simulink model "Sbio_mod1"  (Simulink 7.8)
settings: Solver=ode23t  StartTime=0.0  StopTime=0.5  MinStep=2.9e-4  RelTol=1e-2
PostLoadFcn:
  | openscopes;
undefined symbols (not defined in the file or in its folder): boitier, kg, m, N, porte, poussoir, rad, RootGround, RootPart, s, sigbuilder_block, STL
libraries: mblibv1 x22, fl_lib x16, elec_lib x9, nesl_utility x7

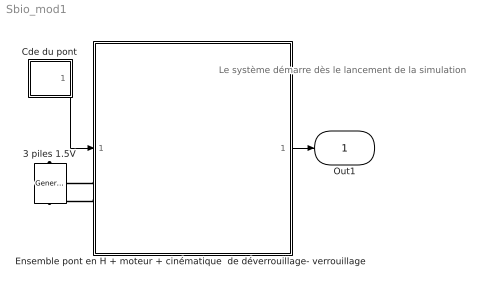
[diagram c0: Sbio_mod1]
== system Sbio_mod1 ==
  note: Le système démarre dès le lancement de la simulation
  3 piles 1.5V : elec_lib/Sources/Generic Battery  Vnom=4.5 V  R1=0.6 Ohm  prm_AH=1  AH=50 hr*A  AH0=50 hr*A  V1=11.5 V  AH1=25 hr*A  prm_R2=1  R2=2e+3 Ohm  LocalVarLogging=[]
  Cde du pont : Subsystem
  Ensemble pont en H + moteur + cinématique  de déverrouillage- verrouillage : Subsystem
  Out1 : Outport
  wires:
  Ensemble pont en H + moteur + cinématique  de déverrouillage- verrouillage/1(Sortie) -> Out1/1
  Cde du pont/1(Out1) -> Ensemble pont en H + moteur + cinématique  de déverrouillage- verrouillage/1(Cdes)
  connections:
  3 piles 1.5V/LConn1 -- Ensemble pont en H + moteur + cinématique  de déverrouillage- verrouillage/LConn1
  3 piles 1.5V/RConn1 -- Ensemble pont en H + moteur + cinématique  de déverrouillage- verrouillage/LConn2

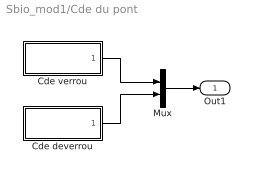
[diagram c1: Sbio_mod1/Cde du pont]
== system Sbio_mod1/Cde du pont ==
  Cde deverrou : Subsystem  Tag=STV Subsys  LoadFcn=sigbuilder_block('load');  StartFcn=sigbuilder_block('start');  StopFcn=sigbuilder_block('stop');  ClipboardFcn=sigbuilder_block('clipboard');
  Cde verrou : Subsystem  Tag=STV Subsys  LoadFcn=sigbuilder_block('load');  StartFcn=sigbuilder_block('start');  StopFcn=sigbuilder_block('stop');  ClipboardFcn=sigbuilder_block('clipboard');
  Mux : Mux  Inputs=2
  Out1 : Outport
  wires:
  Mux/1 -> Out1/1
  Cde verrou/1(Signal 1) -> Mux/1
  Cde deverrou/1(Signal 1) -> Mux/2

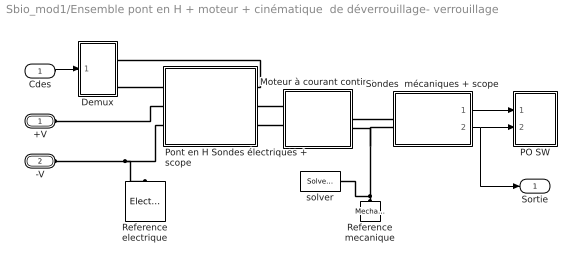
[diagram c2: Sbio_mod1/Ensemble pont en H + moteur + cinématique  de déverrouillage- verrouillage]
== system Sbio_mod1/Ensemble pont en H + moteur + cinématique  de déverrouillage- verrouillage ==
  Cdes : Inport
  Demux : Subsystem
  Moteur à courant continu : Subsystem
  PO SW : Subsystem
  Pont en H Sondes électriques + scope : Subsystem
  Reference electrique : fl_lib/Electrical/Electrical Elements/Electrical Reference  i_Log=off  LocalVarNames=|i  LocalVarDescs=|i  LocalVarLogging=0
  Reference mecanique : fl_lib/Mechanical/Rotational Elements/Mechanical Rotational Reference  t_Log=off  LocalVarNames=|t  LocalVarDescs=|t  LocalVarLogging=0
  Sondes  mécaniques + scope : Subsystem
  solver : nesl_utility/Solver Configuration  PhysicalDomain=network_engine_domain  LeftPortType=input  RightPortType=generic  SubClassName=solver  DoDC=off  ResidualTolerance=1e-9  UseLocalSolver=on  LocalSolverChoice=NE_BACKWARD_EULER_ADVANCER  LocalSolverSampleTime=3e-4  DoFixedCost=on  MaxNonlinIter=5  MaxModeIter=2  LinearAlgebra=Sparse  Accelerate=off  Profile=off  UseLocalSampling=off  DelaysMemoryBudget=1024
  +V : PMIOPort  Port=1  Side=Left
  -V : PMIOPort  Port=2  Side=Left
  Sortie : Outport
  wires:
  Sondes  mécaniques + scope/2(Out2) -> Sortie/1, PO SW/2(In2)
  Sondes  mécaniques + scope/1(Out1) -> PO SW/1(In1)
  Cdes/1 -> Demux/1(I1)
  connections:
  Pont en H Sondes électriques + scope/RConn2 -- +V/RConn1
  -V/RConn1 -- Reference electrique/LConn1 -- Pont en H Sondes électriques + scope/RConn3
  Reference mecanique/LConn1 -- Moteur à courant continu/RConn2 -- Sondes  mécaniques + scope/LConn2 -- solver/RConn1
  Moteur à courant continu/LConn1 -- Pont en H Sondes électriques + scope/LConn2
  Moteur à courant continu/LConn2 -- Pont en H Sondes électriques + scope/LConn3
  Moteur à courant continu/RConn1 -- Sondes  mécaniques + scope/LConn1
  Demux/RConn2 -- Pont en H Sondes électriques + scope/RConn1
  Demux/RConn1 -- Pont en H Sondes électriques + scope/LConn1

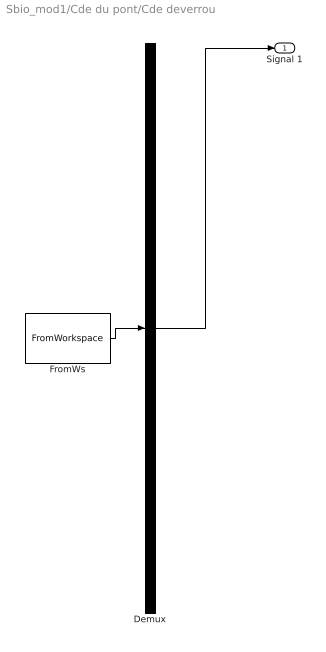
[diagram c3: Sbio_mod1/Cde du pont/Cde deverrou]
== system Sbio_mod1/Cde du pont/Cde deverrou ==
  Demux : Demux  Tag=STV Demux  Outputs=1
  FromWs : FromWorkspace  Tag=STV FromWs  VariableName=tuvar  SampleTime=0  SigBuilderData=DataTag0  VnvData=DataTag1
  Signal 1 : Outport  Tag=STV Outport
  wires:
  Demux/1 -> Signal 1/1
  FromWs/1 -> Demux/1

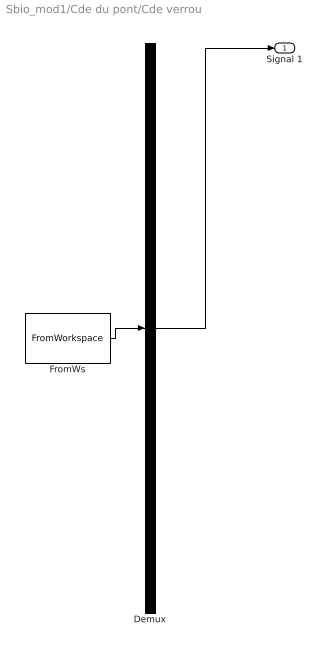
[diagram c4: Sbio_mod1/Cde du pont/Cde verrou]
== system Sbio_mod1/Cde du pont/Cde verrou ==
  Demux : Demux  Tag=STV Demux  Outputs=1
  FromWs : FromWorkspace  Tag=STV FromWs  VariableName=tuvar  SampleTime=0  SigBuilderData=DataTag2  VnvData=DataTag3
  Signal 1 : Outport  Tag=STV Outport
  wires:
  Demux/1 -> Signal 1/1
  FromWs/1 -> Demux/1

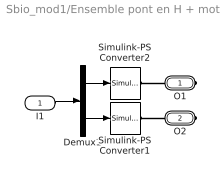
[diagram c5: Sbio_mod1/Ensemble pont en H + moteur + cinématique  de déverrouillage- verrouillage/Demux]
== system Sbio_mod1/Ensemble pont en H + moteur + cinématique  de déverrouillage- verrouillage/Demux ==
  I1 : Inport
  Demux1 : Demux  Outputs=2
  Simulink-PS Converter1 : nesl_utility/Simulink-PS Converter  PhysicalDomain=network_engine_domain  LeftPortType=input  RightPortType=output  SubClassName=ps_input  Unit=1  AffineConversion=off  InputFilterTimeConstant=.01  UdotUserProvided=0
  Simulink-PS Converter2 : nesl_utility/Simulink-PS Converter  PhysicalDomain=network_engine_domain  LeftPortType=input  RightPortType=output  SubClassName=ps_input  Unit=1  AffineConversion=off  InputFilterTimeConstant=.01  UdotUserProvided=0
  O1 : PMIOPort  Port=1  Side=Right
  O2 : PMIOPort  Port=2  Side=Right
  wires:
  Demux1/1 -> Simulink-PS Converter2/1
  Demux1/2 -> Simulink-PS Converter1/1
  I1/1 -> Demux1/1
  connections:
  O1/RConn1 -- Simulink-PS Converter2/RConn1
  O2/RConn1 -- Simulink-PS Converter1/RConn1

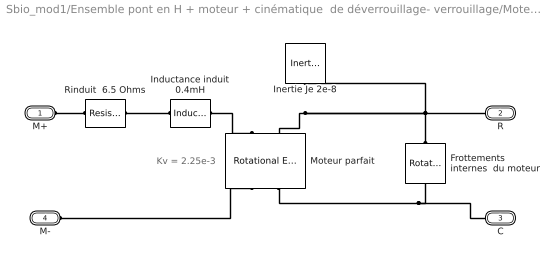
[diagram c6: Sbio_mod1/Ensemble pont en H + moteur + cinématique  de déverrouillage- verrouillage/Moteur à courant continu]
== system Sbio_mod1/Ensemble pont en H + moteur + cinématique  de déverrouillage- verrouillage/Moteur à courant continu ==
  note: Kv = 2.25e-3
  Frottements internes  du moteur : fl_lib/Mechanical/Rotational Elements/Rotational Friction  brkwy_trq=4e-5 N*m  Col_trq=4e-5 N*m  visc_coef=6e-8 N*m/(rad/s)  trans_coef=10 s/rad  vel_thr=1 rad/s  t_Log=off  w_Log=off  LocalVarNames=|t|w  LocalVarDescs=|t|w  LocalVarLogging=[0 0]
  Inductance induit 0.4mH : fl_lib/Electrical/Electrical Elements/Inductor  l=0.4 mH  i0=0 A  r=0 Ohm  g=1e-09 1/Ohm  i_Log=off  v_Log=off  i_L_Log=off  LocalVarNames=|current|voltage|power  LocalVarDescs=|Inductor current (A) |Voltage across inductor (V)|Power (W)  LocalVarLogging=[0 0 0]
  Inertie Je 2e-8 : fl_lib/Mechanical/Rotational Elements/Inertia  inertia=2e-8 kg*m^2  initial_velocity=0 rad/s  t_Log=off  LocalVarNames=|torque|velocity  LocalVarDescs=|Inertia torque (N*m)|Inertia absolute velocity (rad/s)  LocalVarLogging=[0 0]
  Moteur parfait : fl_lib/Electrical/Electrical Elements/Rotational Electromechanical Converter  K=2.25e-3 V/(rad/s)  i_Log=off  v_Log=off  t_Log=off  w_Log=off  LocalVarNames=|current|voltage|power|torque|speed  LocalVarDescs=|Current (A)|Voltage (V)|Power (W)|Torque (Nm)|Angular speed (rad/s)  LocalVarLogging=[0 0 0 0 0]
  Rinduit  6.5 Ohms : fl_lib/Electrical/Electrical Elements/Resistor  Tag=Factory Generic  R=6.5 Ohm  i_Log=off  v_Log=off  LocalVarNames=|current|voltage|power  LocalVarDescs=|Resistor current (A)|Voltage across resistor (V)|Power (W)  LocalVarLogging=[0 0 0]
  M+ : PMIOPort  Port=1  Side=Left
  R : PMIOPort  Port=2  Side=Right
  C : PMIOPort  Port=3  Side=Right
  M- : PMIOPort  Port=4  Side=Left
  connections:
  Moteur parfait/LConn1 -- Inductance induit 0.4mH/RConn1
  M-/RConn1 -- Moteur parfait/RConn1
  M+/RConn1 -- Rinduit  6.5 Ohms/LConn1
  Rinduit  6.5 Ohms/RConn1 -- Inductance induit 0.4mH/LConn1
  Moteur parfait/LConn2 -- Inertie Je 2e-8/LConn1 -- Frottements internes  du moteur/LConn1 -- R/RConn1
  Moteur parfait/RConn2 -- C/RConn1 -- Frottements internes  du moteur/RConn1

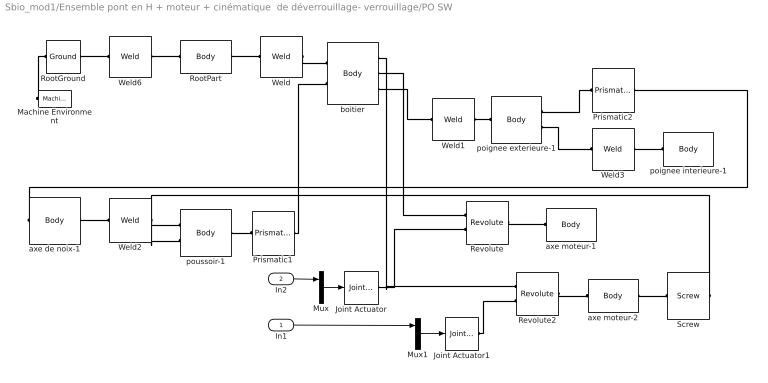
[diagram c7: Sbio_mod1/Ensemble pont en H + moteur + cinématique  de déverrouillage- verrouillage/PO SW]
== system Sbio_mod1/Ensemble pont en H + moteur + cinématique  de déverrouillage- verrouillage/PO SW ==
  In1 : Inport
  In2 : Inport  Port=2
  Joint Actuator : mblibv1/Sensors &  Actuators/Joint Actuator  UpdateFromCAD=off  PhysicalDomain=Mechanical  PortType=blob  ActuationStyle=Motion  AngleUnits=rev  ArcVelocityUnits=rad/s  ArcAccelerationUnits=rad/s^2  CoordPositionUnits=m  VelocityUnits=m/s  AccelerationUnits=m/s^2  ForceUnits=N  TorqueUnits=N*m  ActiveIO=on  Width=3  DialogClass=MechanicalActuatorBlock  Primitive=R1  ReferenceFrame=Absolute (World)
  Joint Actuator1 : mblibv1/Sensors &  Actuators/Joint Actuator  UpdateFromCAD=off  PhysicalDomain=Mechanical  PortType=blob  ActuationStyle=Motion  AngleUnits=rad  ArcVelocityUnits=rad/s  ArcAccelerationUnits=rad/s^2  CoordPositionUnits=m  VelocityUnits=m/s  AccelerationUnits=m/s^2  ForceUnits=N  TorqueUnits=N*m  ActiveIO=on  Width=3  DialogClass=MechanicalActuatorBlock  Primitive=R1  ReferenceFrame=Absolute (World)
  Machine Environment : mblibv1/Bodies/Machine Environment  PortType=env  PhysicalDomain=Mechanical  DialogTemplateClass=MECH.MachineEnvironment  SyncWhenCopied=off  Gravity=[0 -9.81 0]  GravityUnits=m/s^2  GravityAsSignal=off  Dimensionality=Auto-detect  AnalysisType=Forward dynamics  LinearAssemblyTolerance=1e1  LinearAssemblyToleranceUnits=m  AngularAssemblyTolerance=1e1  AngularAssemblyToleranceUnits=rad  ConstraintSolverType=Stabilizing  ConstraintRelTolerance=1e-4  ConstraintAbsTolerance=1e-4  UseRobustSingularityHandling=off  RedundancyAnalysisToleranceType=Specify tolerance  RedundancyAnalysisTolerance=1e-1  StatePerturbationType=Fixed  PerturbationSize=3e-4  VisualizeMachine=on  BodyVisualizationType=Use model default body geometries  BodyColorSelMode=Use model default  DefaultBodyColor=[1 0 0]
  Mux : Mux  Inputs=3
  Mux1 : Mux  Inputs=3
  Prismatic1 : mblibv1/Joints/Prismatic  LConnTagsString=__newl0  RConnTagsString=__newr0  UpdateFromCAD=off  NumSAPorts=0  CutJoint=off  MarkAsCut=off  Primitives=prismatic  PrimitiveProps=P1$World$[0 1 0]$prismatic  DialogClass=JointBlock  P1Axis=[0 1 0]
  Prismatic2 : mblibv1/Joints/Prismatic  LConnTagsString=__newl0  RConnTagsString=__newr0  UpdateFromCAD=off  NumSAPorts=0  CutJoint=off  MarkAsCut=off  Primitives=prismatic  PrimitiveProps=P1$World$[0 1 0]$prismatic  DialogClass=JointBlock  P1Axis=[0 1 0]
  Revolute : mblibv1/Joints/Revolute  LConnTagsString=__newl0|SA1  RConnTagsString=__newr0  UpdateFromCAD=on  PMImportedID=axe moteur-1:-:porte-1  NumSAPorts=1  CutJoint=off  MarkAsCut=off  Primitives=prismatic  PrimitiveProps=R1$World$[0,1,0]$revolute  DialogClass=JointBlock  R1Axis=[0,1,0]
  Revolute2 : mblibv1/Joints/Revolute  LConnTagsString=__newl0|SA1  RConnTagsString=__newr0  UpdateFromCAD=on  NumSAPorts=1  CutJoint=off  MarkAsCut=off  Primitives=prismatic  PrimitiveProps=R1$World$[0,1,0]$revolute  DialogClass=JointBlock  R1Axis=[0,1,0]
  RootGround : mblibv1/Bodies/Ground  UpdateFromCAD=on  PMImportedID=RootGround  LeftPortType=env  RightPortType=workingframe  PhysicalDomain=Mechanical  DialogClass=GroundBlock  CoordPosition=[-0.0761581,-0.00065379,-0.00321688]  CoordPositionUnits=m  StateVectorMgrId=0  MachineId=[1 0]  ShowEnvPort=on
  RootPart : mblibv1/Bodies/Body  LConnTagsString=CS3  RConnTagsString=CS2  UpdateFromCAD=on  PMImportedID=RootPart  DialogClass=MechanicalBodyBlock  Mass=0  MassUnits=kg  InertiaUnits=kg*m^2  Inertia=[0,0,0;0,0,0;0,0,0]  Shape=Cylinder  ShapeDims=[1 1]  ShapeUnits=m  ShapeUse=false  Density=1  DensityUnits=kg/m^3  DensityUse=false  GraphicsMode=MACHINE_DEFAULT  BodyColorSelMode=MACHINE_DEFAULT  BodyColor=[1 0 0]  AttachedToCS=CS1  CG=Right$CG$[-0.0761581 -0.00065379 -0.00321688]$WORLD$WORLD$m$[1 0 0;0 1 0;0 0 1]$3x3 Transform$rad$WORLD$false$RootPart::CG(AUTOGEN)  WorkingFrames=Right$CS1$[0 0 0]$WORLD$WORLD$m$[1 0 0;0 1 0;0 0 1]$3x3 Transform$rad$WORLD$false$RootPart::CS1(AUTOGEN)#Right$CS2$[-0.077666 -3.78754e-005 -0.00401674]$WORLD$WORLD$m$[1 0 0;0 1 0;0 0 1]$3x3 Transform$rad$WORLD$true$RootPart:-:porte-1::RootPart(AUTOGEN)#Left$CS3$[-0.0761581 -0.00065379 -0.00321688]$WORLD$WORLD$m$[1 0 0;0 1 0;0 0 1]$3x3 Transform$rad$WORLD$true$RootGround:-:RootPart::RootPart(AUTOG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  CGPos=[-0.0761581 -0.00065379 -0.00321688]  CGRot=[1 0 0;0 1 0;0 0 1]  CS0Pos=[]  CS0Rot=[]  CS1Pos=[0 0 0]  CS1Rot=[1 0 0;0 1 0;0 0 1]  CS2Pos=[-0.077666 -3.78754e-005 -0.00401674]  CS2Rot=[1 0 0;0 1 0;0 0 1]  CS3Pos=[-0.0761581 -0.00065379 -0.00321688]  CS3Rot=[1 0 0;0 1 0;0 0 1]  CS4Pos=[]  CS4Rot=[]  CS5Pos=[]  CS5Rot=[]  CS6Pos=[]  CS6Rot=[]  CS7Pos=[]  CS7Rot=[]  CS8Pos=[]  CS8Rot=[]  CS9Pos=[]  CS9Rot=[]  CS10Pos=[]  CS10Rot=[]  CS11Pos=[]  CS11Rot=[]  CS12Pos=[]  CS12Rot=[]  CS13Pos=[]  CS13Rot=[]  CS14Pos=[]  CS14Rot=[]  CS15Pos=[]  CS15Rot=[]  CS16Pos=[]  CS16Rot=[]  CS17Pos=[]  CS17Rot=[]  CS18Pos=[]  CS18Rot=[]  CS19Pos=[]  CS19Rot=[]  CS20Pos=[]  CS20Rot=[]
  Screw : mblibv1/Joints/Screw  LConnTagsString=__newl0  RConnTagsString=__newr0  UpdateFromCAD=off  NumSAPorts=0  CutJoint=off  MarkAsCut=off  Primitives=prismatic  PrimitiveProps=R1$World$[0 1 0]$revolute  DialogClass=ScrewJointBlock  Pitch=2  Units=mm  R1Axis=[0 1 0]
  Weld : mblibv1/Joints/Weld  LConnTagsString=__newl0  RConnTagsString=__newr0  UpdateFromCAD=on  PMImportedID=RootPart:-:porte-1  NumSAPorts=0  CutJoint=off  MarkAsCut=off  Primitives=weld  PrimitiveProps=W$WORLD$[0.57735,0.57735,0.57735]$weld  DialogClass=JointBlock  WAxis=[0.57735,0.57735,0.57735]
  Weld1 : mblibv1/Joints/Weld  LConnTagsString=__newl0  RConnTagsString=__newr0  UpdateFromCAD=on  NumSAPorts=0  CutJoint=off  MarkAsCut=off  Primitives=weld  PrimitiveProps=W$WORLD$[0.57735,0.57735,0.57735]$weld  DialogClass=JointBlock  WAxis=[0.57735,0.57735,0.57735]
  Weld2 : mblibv1/Joints/Weld  LConnTagsString=__newl0  RConnTagsString=__newr0  UpdateFromCAD=on  NumSAPorts=0  CutJoint=off  MarkAsCut=off  Primitives=weld  PrimitiveProps=W$World$[0.57735,0.57735,0.57735]$weld  DialogClass=JointBlock  WAxis=[0.57735,0.57735,0.57735]
  Weld3 : mblibv1/Joints/Weld  LConnTagsString=__newl0  RConnTagsString=__newr0  UpdateFromCAD=on  PMImportedID=poignee exterieure-1:-:poignee interieure-1  NumSAPorts=0  CutJoint=off  MarkAsCut=off  Primitives=weld  PrimitiveProps=W$WORLD$[0.57735,0.57735,0.57735]$weld  DialogClass=JointBlock  WAxis=[0.57735,0.57735,0.57735]
  Weld6 : mblibv1/Joints/Weld  LConnTagsString=__newl0  RConnTagsString=__newr0  UpdateFromCAD=on  PMImportedID=RootGround:-:RootPart  NumSAPorts=0  CutJoint=off  MarkAsCut=off  Primitives=weld  PrimitiveProps=W$WORLD$[0.57735,0.57735,0.57735]$weld  DialogClass=JointBlock  WAxis=[0.57735,0.57735,0.57735]
  axe de noix-1 : mblibv1/Bodies/Body  LConnTagsString=CS3  RConnTagsString=CS2  UpdateFromCAD=on  PMImportedID=axe de noix-1  DialogClass=MechanicalBodyBlock  Mass=0.00163609  MassUnits=kg  InertiaUnits=kg*m^2  Inertia=[4.0118e-009,4.23855e-014,6.10726e-014;4.23855e-014,2.95718e-008,-1.28692e-014;6.10726e-014,-1.28692e-014,2.95718e-008]  Shape=Cylinder  ShapeDims=[1 1]  ShapeUnits=m  ShapeUse=false  Density=1  DensityUnits=kg/m^3  DensityUse=false  GraphicsMode=GFXFILE  GraphicsFileName=STL\axe de noix-1.STL  BodyColorSelMode=COLORPALETTE  BodyColor=[0 1 0]  AttachedToCS=CS1  CG=Right$CG$[-0.0711604 0.0108855 -3.81612e-009]$WORLD$WORLD$m$[0 0.110851 0.993837;1 0 0;0 0.993837 -0.110851]$3x3 Transform$rad$WORLD$false$axe de noix-1::CG(AUTOGEN)  WorkingFrames=Right$CS1$[-0.0711604 0.00328332 0]$WORLD$WORLD$m$[0 0.110851 0.993837;1 0 0;0 0.993837 -0.110851]$3x3 Transform$rad$WORLD$false$axe de noix-1::CS1(AUTOGEN)#Right$CS2$[-0.0711604 0.0108855 -3.81612e-009]$WORLD$WORLD$m$[1 0 0;0 1 0;0 0 1]$3x3 Transform$rad$WORLD$true$axe de noix-1:-:poussoir-1::axe de noix-1(AUTOGEN)#Left$CS3$[-0.0711604 0.00457656 0]$World$World$m$[1 0 0;0 1 0;0 0 1]$3x3 Transform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  CGPos=[-0.0711604 0.0108855 -3.81612e-009]  CGRot=[0 0.110851 0.993837;1 0 0;0 0.993837 -0.110851]  CS0Pos=[]  CS0Rot=[]  CS1Pos=[-0.0711604 0.00328332 0]  CS1Rot=[0 0.110851 0.993837;1 0 0;0 0.993837 -0.110851]  CS2Pos=[-0.0711604 0.0108855 -3.81612e-009]  CS2Rot=[1 0 0;0 1 0;0 0 1]  CS3Pos=[-0.0711604 0.00457656 0]  CS3Rot=[1 0 0;0 1 0;0 0 1]  CS4Pos=[-0.0675087 0.0349848 -0.00412076]  CS4Rot=[1 0 0;0 1 0;0 0 1]  CS5Pos=[]  CS5Rot=[]  CS6Pos=[]  CS6Rot=[]  CS7Pos=[]  CS7Rot=[]  CS8Pos=[]  CS8Rot=[]  CS9Pos=[]  CS9Rot=[]  CS10Pos=[]  CS10Rot=[]  CS11Pos=[]  CS11Rot=[]  CS12Pos=[]  CS12Rot=[]  CS13Pos=[]  CS13Rot=[]  CS14Pos=[]  CS14Rot=[]  CS15Pos=[]  CS15Rot=[]  CS16Pos=[]  CS16Rot=[]  CS17Pos=[]  CS17Rot=[]  CS18Pos=[]  CS18Rot=[]  CS19Pos=[]  CS19Rot=[]  CS20Pos=[]  CS20Rot=[]
  axe moteur-1 : mblibv1/Bodies/Body  LConnTagsString=CS3  UpdateFromCAD=on  PMImportedID=axe moteur-1  DialogClass=MechanicalBodyBlock  Mass=5  MassUnits=g  InertiaUnits=kg*m^2  Inertia=[2.93484e-010,5.6457e-012,-1.21489e-012;5.6457e-012,9.47861e-011,6.78023e-012;-1.21489e-012,6.78023e-012,2.93562e-010]  Shape=Cylinder  ShapeDims=[1 1]  ShapeUnits=m  ShapeUse=false  Density=1  DensityUnits=kg/m^3  DensityUse=false  GraphicsMode=GFXFILE  GraphicsFileName=STL\axe moteur-1.STL  BodyColorSelMode=COLORPALETTE  BodyColor=[1 0 0]  AttachedToCS=CS1  CG=Right$CG$[-0.0675804 0.0226495 0.000154618]$WORLD$WORLD$m$[-0.968237 0 -0.250035;0 1 0;0.250035 0 -0.968237]$3x3 Transform$rad$WORLD$false$axe moteur-1::CG(AUTOGEN)  WorkingFrames=Right$CS1$[-0.0713109 0.0213931 -0.012834]$WORLD$WORLD$m$[-0.968237 0 -0.250035;0 1 0;0.250035 0 -0.968237]$3x3 Transform$rad$WORLD$false$axe moteur-1::CS1(AUTOGEN)#Left$CS3$[-0.0675633 0.0260507 0.000120417]$WORLD$WORLD$m$[1 0 0;0 1 0;0 0 1]$3x3 Transform$rad$WORLD$true$axe moteur-1:-:porte-1::axe moteur-1(AUTOGEN)  CGPos=[-0.0675804 0.0226495 0.000154618]  CGRot=[-0.968237 0 -0.250035;0 1 0;0.250035 0 -0.968237]  CS0Pos=[]  CS0Rot=[]  CS1Pos=[-0.0713109 0.0213931 -0.012834]  CS1Rot=[-0.968237 0 -0.250035;0 1 0;0.250035 0 -0.968237]  CS2Pos=[]  CS2Rot=[]  CS3Pos=[-0.0675633 0.0260507 0.000120417]  CS3Rot=[1 0 0;0 1 0;0 0 1]  CS4Pos=[]  CS4Rot=[]  CS5Pos=[]  CS5Rot=[]  CS6Pos=[]  CS6Rot=[]  CS7Pos=[]  CS7Rot=[]  CS8Pos=[]  CS8Rot=[]  CS9Pos=[]  CS9Rot=[]  CS10Pos=[]  CS10Rot=[]  CS11Pos=[]  CS11Rot=[]  CS12Pos=[]  CS12Rot=[]  CS13Pos=[]  CS13Rot=[]  CS14Pos=[]  CS14Rot=[]  CS15Pos=[]  CS15Rot=[]  CS16Pos=[]  CS16Rot=[]  CS17Pos=[]  CS17Rot=[]  CS18Pos=[]  CS18Rot=[]  CS19Pos=[]  CS19Rot=[]  CS20Pos=[]  CS20Rot=[]
  axe moteur-2 : mblibv1/Bodies/Body  LConnTagsString=CS3  RConnTagsString=CS2  UpdateFromCAD=on  DialogClass=MechanicalBodyBlock  Mass=1  MassUnits=g  InertiaUnits=kg*m^2  Inertia=[2.93484e-010,5.6457e-012,-1.21489e-012;5.6457e-012,9.47861e-011,6.78023e-012;-1.21489e-012,6.78023e-012,2.93562e-010]  Shape=Cylinder  ShapeDims=[1 1]  ShapeUnits=m  ShapeUse=false  Density=1  DensityUnits=kg/m^3  DensityUse=false  GraphicsMode=GFXFILE  GraphicsFileName=STL\axe moteur-1.STL  BodyColorSelMode=COLORPALETTE  BodyColor=[1 0 0]  AttachedToCS=CS1  CG=Right$CG$[-0.0675804 0.0226495 0.000154618]$WORLD$WORLD$m$[-0.968237 0 -0.250035;0 1 0;0.250035 0 -0.968237]$3x3 Transform$rad$WORLD$false$none  WorkingFrames=Right$CS1$[-0.0713109 0.0213931 -0.012834]$WORLD$WORLD$m$[-0.968237 0 -0.250035;0 1 0;0.250035 0 -0.968237]$3x3 Transform$rad$WORLD$false$none#Right$CS2$[-0.0675804 0.0226495 0.000154618]$WORLD$WORLD$m$[1 0 0;0 1 0;0 0 1]$3x3 Transform$rad$WORLD$true$none#Left$CS3$[-0.0675633 0.0260507 0.000120417]$WORLD$WORLD$m$[1 0 0;0 1 0;0 0 1]$3x3 Transform$rad$WORLD$true$none  CGPos=[-0.0675804 0.0226495 0.000154618]  CGRot=[-0.968237 0 -0.250035;0 1 0;0.250035 0 -0.968237]  CS0Pos=[]  CS0Rot=[]  CS1Pos=[-0.0713109 0.0213931 -0.012834]  CS1Rot=[-0.968237 0 -0.250035;0 1 0;0.250035 0 -0.968237]  CS2Pos=[-0.0675804 0.0226495 0.000154618]  CS2Rot=[1 0 0;0 1 0;0 0 1]  CS3Pos=[-0.0675633 0.0260507 0.000120417]  CS3Rot=[1 0 0;0 1 0;0 0 1]  CS4Pos=[]  CS4Rot=[]  CS5Pos=[]  CS5Rot=[]  CS6Pos=[]  CS6Rot=[]  CS7Pos=[]  CS7Rot=[]  CS8Pos=[]  CS8Rot=[]  CS9Pos=[]  CS9Rot=[]  CS10Pos=[]  CS10Rot=[]  CS11Pos=[]  CS11Rot=[]  CS12Pos=[]  CS12Rot=[]  CS13Pos=[]  CS13Rot=[]  CS14Pos=[]  CS14Rot=[]  CS15Pos=[]  CS15Rot=[]  CS16Pos=[]  CS16Rot=[]  CS17Pos=[]  CS17Rot=[]  CS18Pos=[]  CS18Rot=[]  CS19Pos=[]  CS19Rot=[]  CS20Pos=[]  CS20Rot=[]
  boitier : mblibv1/Bodies/Body  LConnTagsString=CS2|CS4  RConnTagsString=CS3|CS5|CS6  UpdateFromCAD=on  PMImportedID=porte-1  DialogClass=MechanicalBodyBlock  Mass=0.0422218  MassUnits=kg  InertiaUnits=kg*m^2  Inertia=[9.81362e-005,-9.63885e-006,-9.60739e-007;-9.63885e-006,1.8326e-005,-3.01233e-006;-9.60739e-007,-3.01233e-006,0.000115438]  Shape=Cylinder  ShapeDims=[1 1]  ShapeUnits=m  ShapeUse=false  Density=1  DensityUnits=kg/m^3  DensityUse=false  GraphicsMode=GFXFILE  GraphicsFileName=STL\boitier-1.STL  BodyColorSelMode=COLORPALETTE  BodyColor=[0.75686 0.86667 0.77647]  AttachedToCS=CS1  CG=Right$CG$[-0.077666 -3.78754e-005 -0.00401674]$WORLD$WORLD$m$[1 0 0;0 1 0;0 0 1]$3x3 Transform$rad$WORLD$false$porte-1::CG(AUTOGEN)  WorkingFrames=Right$CS1$[0 0 0]$WORLD$WORLD$m$[1 0 0;0 1 0;0 0 1]$3x3 Transform$rad$WORLD$false$porte-1::CS1(AUTOGEN)#Left$CS2$[-0.077666 -3.78754e-005 -0.00401674]$WORLD$WORLD$m$[1 0 0;0 1 0;0 0 1]$3x3 Transform$rad$WORLD$true$RootPart:-:porte-1::porte-1(AUTOGEN)#Right$CS3$[-0.0675087 0.0349848 -0.00412076]$WORLD$WORLD$m$[1 0 0;0 1 0;0 0 1]$3x3 Transform$rad$WORLD$true$axe de noix-1:-:porte-1::porte-1(AUTOGEN)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  CGPos=[-0.077666 -3.78754e-005 -0.00401674]  CGRot=[1 0 0;0 1 0;0 0 1]  CS0Pos=[]  CS0Rot=[]  CS1Pos=[0 0 0]  CS1Rot=[1 0 0;0 1 0;0 0 1]  CS2Pos=[-0.077666 -3.78754e-005 -0.00401674]  CS2Rot=[1 0 0;0 1 0;0 0 1]  CS3Pos=[-0.0675087 0.0349848 -0.00412076]  CS3Rot=[1 0 0;0 1 0;0 0 1]  CS4Pos=[-0.0606604 0.0186833 0.0035]  CS4Rot=[1 0 0;0 1 0;0 0 1]  CS5Pos=[-0.0675633 0.0260507 0.000120417]  CS5Rot=[1 0 0;0 1 0;0 0 1]  CS6Pos=[-0.0711604 -0.00542344 -0.0055]  CS6Rot=[1 0 0;0 1 0;0 0 1]  CS7Pos=[]  CS7Rot=[]  CS8Pos=[]  CS8Rot=[]  CS9Pos=[]  CS9Rot=[]  CS10Pos=[]  CS10Rot=[]  CS11Pos=[]  CS11Rot=[]  CS12Pos=[]  CS12Rot=[]  CS13Pos=[]  CS13Rot=[]  CS14Pos=[]  CS14Rot=[]  CS15Pos=[]  CS15Rot=[]  CS16Pos=[]  CS16Rot=[]  CS17Pos=[]  CS17Rot=[]  CS18Pos=[]  CS18Rot=[]  CS19Pos=[]  CS19Rot=[]  CS20Pos=[]  CS20Rot=[]
  poignee exterieure-1 : mblibv1/Bodies/Body  LConnTagsString=CS4  RConnTagsString=CS2|CS3  UpdateFromCAD=on  PMImportedID=poignee exterieure-1  DialogClass=MechanicalBodyBlock  Mass=0.00460447  MassUnits=kg  InertiaUnits=kg*m^2  Inertia=[1.37365e-006,-1.46016e-010,-5.00265e-010;-1.46016e-010,1.37543e-006,6.14988e-009;-5.00265e-010,6.14988e-009,1.04136e-007]  Shape=Cylinder  ShapeDims=[1 1]  ShapeUnits=m  ShapeUse=false  Density=1  DensityUnits=kg/m^3  DensityUse=false  GraphicsMode=GFXFILE  GraphicsFileName=STL\poignee exterieure-1.STL  BodyColorSelMode=COLORPALETTE  BodyColor=[0.67843 0.92157 1]  AttachedToCS=CS1  CG=Right$CG$[-0.0711604 -0.0054856 -0.0215575]$WORLD$WORLD$m$[0.996714 0.0810068 0;-0.0810068 0.996714 0;0 0 1]$3x3 Transform$rad$WORLD$false$poignee exterieure-1::CG(AUTOGEN)  WorkingFrames=Right$CS1$[0.00020547 -0.0057823 -0.0015]$WORLD$WORLD$m$[0.996714 0.0810068 0;-0.0810068 0.996714 0;0 0 1]$3x3 Transform$rad$WORLD$false$poignee exterieure-1::CS1(AUTOGEN)#Right$CS2$[-0.0711604 0.00457656 0]$WORLD$WORLD$m$[1 0 0;0 1 0;0 0 1]$3x3 Transform$rad$WORLD$true$axe de noix-1:-:poignee exterieure-1::poignee exterieure-1(AUTOGEN)#Right$CS3$[-0.0711604 -0.00542344 -0.0681035]$WORLD$WORLD$m$[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  CGPos=[-0.0711604 -0.0054856 -0.0215575]  CGRot=[0.996714 0.0810068 0;-0.0810068 0.996714 0;0 0 1]  CS0Pos=[]  CS0Rot=[]  CS1Pos=[0.00020547 -0.0057823 -0.0015]  CS1Rot=[0.996714 0.0810068 0;-0.0810068 0.996714 0;0 0 1]  CS2Pos=[-0.0711604 0.00457656 0]  CS2Rot=[1 0 0;0 1 0;0 0 1]  CS3Pos=[-0.0711604 -0.00542344 -0.0681035]  CS3Rot=[1 0 0;0 1 0;0 0 1]  CS4Pos=[-0.0711604 -0.00542344 -0.0055]  CS4Rot=[1 0 0;0 1 0;0 0 1]  CS5Pos=[]  CS5Rot=[]  CS6Pos=[]  CS6Rot=[]  CS7Pos=[]  CS7Rot=[]  CS8Pos=[]  CS8Rot=[]  CS9Pos=[]  CS9Rot=[]  CS10Pos=[]  CS10Rot=[]  CS11Pos=[]  CS11Rot=[]  CS12Pos=[]  CS12Rot=[]  CS13Pos=[]  CS13Rot=[]  CS14Pos=[]  CS14Rot=[]  CS15Pos=[]  CS15Rot=[]  CS16Pos=[]  CS16Rot=[]  CS17Pos=[]  CS17Rot=[]  CS18Pos=[]  CS18Rot=[]  CS19Pos=[]  CS19Rot=[]  CS20Pos=[]  CS20Rot=[]
  poignee interieure-1 : mblibv1/Bodies/Body  LConnTagsString=CS2  UpdateFromCAD=on  PMImportedID=poignee interieure-1  DialogClass=MechanicalBodyBlock  Mass=0.00860191  MassUnits=kg  InertiaUnits=kg*m^2  Inertia=[2.46815e-006,-2.8953e-007,-1.29467e-007;-2.8953e-007,2.51954e-006,5.61647e-008;-1.29467e-007,5.61647e-008,1.13589e-006]  Shape=Cylinder  ShapeDims=[1 1]  ShapeUnits=m  ShapeUse=false  Density=1  DensityUnits=kg/m^3  DensityUse=false  GraphicsMode=GFXFILE  GraphicsFileName=STL\poignee interieure-1.STL  BodyColorSelMode=COLORPALETTE  BodyColor=[1 0.69412 0.39216]  AttachedToCS=CS1  CG=Right$CG$[-0.0724516 -0.00458394 0.00973531]$WORLD$WORLD$m$[1 7.44962e-012 1.63898e-011;-7.44962e-012 1 -1.13591e-010;-1.63898e-011 1.13591e-010 1]$3x3 Transform$rad$WORLD$false$poignee interieure-1::CG(AUTOGEN)  WorkingFrames=Right$CS1$[0 0 -0.0013]$WORLD$WORLD$m$[1 7.44962e-012 1.63898e-011;-7.44962e-012 1 -1.13591e-010;-1.63898e-011 1.13591e-010 1]$3x3 Transform$rad$WORLD$false$poignee interieure-1::CS1(AUTOGEN)#Left$CS2$[-0.0711604 -0.00542344 -0.0681035]$WORLD$WORLD$m$[1 0 0;0 1 0;0 0 1]$3x3 Transform$rad$WORLD$true$poignee exterieure-1:-:poignee interieure-1::poignee interieure-1(AUTOGEN)  CGPos=[-0.0724516 -0.00458394 0.00973531]  CGRot=[1 7.44962e-012 1.63898e-011;-7.44962e-012 1 -1.13591e-010;-1.63898e-011 1.13591e-010 1]  CS0Pos=[]  CS0Rot=[]  CS1Pos=[0 0 -0.0013]  CS1Rot=[1 7.44962e-012 1.63898e-011;-7.44962e-012 1 -1.13591e-010;-1.63898e-011 1.13591e-010 1]  CS2Pos=[-0.0711604 -0.00542344 -0.0681035]  CS2Rot=[1 0 0;0 1 0;0 0 1]  CS3Pos=[]  CS3Rot=[]  CS4Pos=[]  CS4Rot=[]  CS5Pos=[]  CS5Rot=[]  CS6Pos=[]  CS6Rot=[]  CS7Pos=[]  CS7Rot=[]  CS8Pos=[]  CS8Rot=[]  CS9Pos=[]  CS9Rot=[]  CS10Pos=[]  CS10Rot=[]  CS11Pos=[]  CS11Rot=[]  CS12Pos=[]  CS12Rot=[]  CS13Pos=[]  CS13Rot=[]  CS14Pos=[]  CS14Rot=[]  CS15Pos=[]  CS15Rot=[]  CS16Pos=[]  CS16Rot=[]  CS17Pos=[]  CS17Rot=[]  CS18Pos=[]  CS18Rot=[]  CS19Pos=[]  CS19Rot=[]  CS20Pos=[]  CS20Rot=[]
  poussoir-1 : mblibv1/Bodies/Body  LConnTagsString=CS2|CS3  RConnTagsString=CS4  UpdateFromCAD=on  PMImportedID=poussoir-1  DialogClass=MechanicalBodyBlock  Mass=0.000364483  MassUnits=kg  InertiaUnits=kg*m^2  Inertia=[1.07048e-008,-7.00376e-009,5.05517e-013;-7.00376e-009,1.80137e-008,-1.71926e-011;5.05517e-013,-1.71926e-011,2.65385e-008]  Shape=Cylinder  ShapeDims=[1 1]  ShapeUnits=m  ShapeUse=false  Density=1  DensityUnits=kg/m^3  DensityUse=false  GraphicsMode=GFXFILE  GraphicsFileName=STL\poussoir-1.STL  BodyColorSelMode=COLORPALETTE  BodyColor=[1 1 0]  AttachedToCS=CS1  CG=Right$CG$[-0.075864 0.0263694 0.00049425]$WORLD$WORLD$m$[0 -1 0;1 0 0;0 0 1]$3x3 Transform$rad$WORLD$false$poussoir-1::CG(AUTOGEN)  WorkingFrames=Right$CS1$[-0.0461604 -0.104076 -0.0025]$WORLD$WORLD$m$[0 -1 0;1 0 0;0 0 1]$3x3 Transform$rad$WORLD$false$poussoir-1::CS1(AUTOGEN)#Left$CS2$[-0.0711604 0.0108855 -3.81612e-009]$WORLD$WORLD$m$[1 0 0;0 1 0;0 0 1]$3x3 Transform$rad$WORLD$true$axe de noix-1:-:poussoir-1::poussoir-1(AUTOGEN)#Left$CS3$[-0.0675804 0.0226495 0.000154618]$WORLD$WORLD$m$[1 0 0;0 1 0;0 0 1]$3x3 Transform$rad$WORLD$true$axe m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  CGPos=[-0.075864 0.0263694 0.00049425]  CGRot=[0 -1 0;1 0 0;0 0 1]  CS0Pos=[]  CS0Rot=[]  CS1Pos=[-0.0461604 -0.104076 -0.0025]  CS1Rot=[0 -1 0;1 0 0;0 0 1]  CS2Pos=[-0.0711604 0.0108855 -3.81612e-009]  CS2Rot=[1 0 0;0 1 0;0 0 1]  CS3Pos=[-0.0675804 0.0226495 0.000154618]  CS3Rot=[1 0 0;0 1 0;0 0 1]  CS4Pos=[-0.0606604 0.0186833 0.0035]  CS4Rot=[1 0 0;0 1 0;0 0 1]  CS5Pos=[]  CS5Rot=[]  CS6Pos=[]  CS6Rot=[]  CS7Pos=[]  CS7Rot=[]  CS8Pos=[]  CS8Rot=[]  CS9Pos=[]  CS9Rot=[]  CS10Pos=[]  CS10Rot=[]  CS11Pos=[]  CS11Rot=[]  CS12Pos=[]  CS12Rot=[]  CS13Pos=[]  CS13Rot=[]  CS14Pos=[]  CS14Rot=[]  CS15Pos=[]  CS15Rot=[]  CS16Pos=[]  CS16Rot=[]  CS17Pos=[]  CS17Rot=[]  CS18Pos=[]  CS18Rot=[]  CS19Pos=[]  CS19Rot=[]  CS20Pos=[]  CS20Rot=[]
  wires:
  Mux/1 -> Joint Actuator/1
  In1/1 -> Mux1/1
  Mux1/1 -> Joint Actuator1/1
  In2/1 -> Mux/1
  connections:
  axe de noix-1/RConn1 -- Weld2/RConn1
  Weld2/LConn1 -- poussoir-1/LConn1
  RootGround/LConn1 -- Machine Environment/RConn1
  Revolute/RConn1 -- axe moteur-1/LConn1
  boitier/RConn3 -- Weld1/LConn1
  Weld1/RConn1 -- poignee exterieure-1/LConn1
  RootGround/RConn1 -- Weld6/LConn1
  Weld6/RConn1 -- RootPart/LConn1
  RootPart/RConn1 -- Weld/LConn1
  Weld/RConn1 -- boitier/LConn1
  poignee exterieure-1/RConn2 -- Weld3/LConn1
  Weld3/RConn1 -- poignee interieure-1/LConn1
  Screw/RConn1 -- poussoir-1/LConn2
  Revolute2/RConn1 -- axe moteur-2/LConn1
  Joint Actuator1/RConn1 -- Revolute2/LConn2
  boitier/RConn1 -- Revolute2/LConn1
  boitier/RConn2 -- Revolute/LConn1
  Joint Actuator/RConn1 -- Revolute/LConn2
  axe moteur-2/RConn1 -- Screw/LConn1
  Prismatic1/RConn1 -- boitier/LConn2
  poussoir-1/RConn1 -- Prismatic1/LConn1
  Prismatic2/RConn1 -- poignee exterieure-1/RConn1
  axe de noix-1/LConn1 -- Prismatic2/LConn1

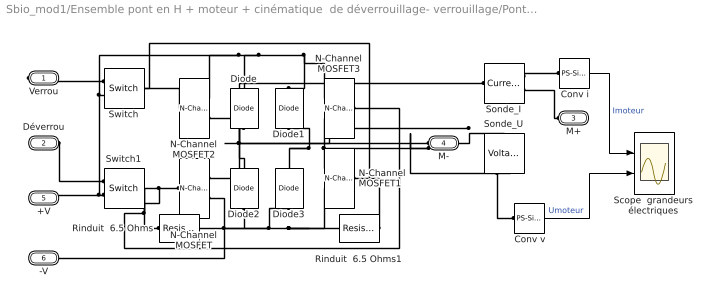
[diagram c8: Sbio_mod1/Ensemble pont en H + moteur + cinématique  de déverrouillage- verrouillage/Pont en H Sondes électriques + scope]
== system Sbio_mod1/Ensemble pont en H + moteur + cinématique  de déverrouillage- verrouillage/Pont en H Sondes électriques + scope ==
  " Conv i" : nesl_utility/PS-Simulink Converter  PhysicalDomain=network_engine_domain  LeftPortType=input  RightPortType=output  SubClassName=ps_output  Unit=1  AffineConversion=off
  " Conv v" : nesl_utility/PS-Simulink Converter  PhysicalDomain=network_engine_domain  LeftPortType=input  RightPortType=output  SubClassName=ps_output  Unit=1  AffineConversion=off
  Diode{,1..3} (4 alike) : elec_lib/Semiconductor Devices/Diode  ModelType=1  Vf=0.6 V  Ron=0.3 Ohm  Goff=1e-8 S  Rz=0.3 Ohm  Vz=50 V  C_PWL=5 pF  prmExp=1  I12=[ 0.07 1.5 ] A  V12=[ 0.7 0.8 ] V  I1=0.07 A  V1=0.7 V  RS=0.01 Ohm  IS=1e-14 A  Tmeas=25 C  ec=1  BV=Inf V  C_param=1  CJ0=5 pF  VJ=1 V  Mgrad=0.5  Vvec=[ 0.1 10 100 ] V  Cvec=[ 3.5 1 0.4 ] pF  FC=0.5  T_param=1  IS_T2=1.25e-7 A  I1_T2=0.245 A  V1_T2=0.5 V  Tmeas2=125 C  EG_param=1  EG=1.11 eV  XTI_param=1  XTI=3  dBVdT=0 V/K  Tdevice=25 C  LocalVarLogging=[]  Rth=[ 0 10 ] K/W  thermal_mass_parameterization=1  thermal_mass=[ 0 1 ] J/K  thermal_time_constant=[ 0 10 ] s  thermal_mass_initial_temperatures=[ 25 25 ] C
  N-Channel MOSFET : elec_lib/Semiconductor Devices/N-Channel MOSFET  parameterization=2  prmDatasheet=1  prmEquCoeff=1  Beta=5 A/V^2  Rds=0.025 Ohm  Id=6 A  Vgs=12 V  Vth=0.2 V  lam=0 1/V  Tmeas=25 C  RS=1e-4 Ohm  RD=0.01 Ohm  C_param=1  C_GS=270 pF  C_GD=80 pF  C_iss=350 pF  C_rss=80 pF  dVth_dT=-6 mV/K  Rds_T2=0.037 Ohm  Tmeas2=125 C  BEXDatasheet=-1.5  BEXEquCoeff=-1.5  TdeviceDatasheet=25 C  TdeviceEquCoeff=25 C  LocalVarLogging=[]  Rth=[ 0 10 ] K/W  thermal_mass_parameterization=1  thermal_mass=[ 0 1 ] J/K  thermal_time_constant=[ 0 10 ] s  thermal_mass_initial_temperatures=[ 25 25 ] C
  N-Channel MOSFET1 : elec_lib/Semiconductor Devices/N-Channel MOSFET  parameterization=2  prmDatasheet=1  prmEquCoeff=1  Beta=5 A/V^2  Rds=0.025 Ohm  Id=6 A  Vgs=10 V  Vth=0.3 V  lam=0 1/V  Tmeas=25 C  RS=1e-4 Ohm  RD=0.01 Ohm  C_param=1  C_GS=270 pF  C_GD=80 pF  C_iss=350 pF  C_rss=80 pF  dVth_dT=-6 mV/K  Rds_T2=0.037 Ohm  Tmeas2=125 C  BEXDatasheet=-1.5  BEXEquCoeff=-1.5  TdeviceDatasheet=25 C  TdeviceEquCoeff=25 C  LocalVarLogging=[]  Rth=[ 0 10 ] K/W  thermal_mass_parameterization=1  thermal_mass=[ 0 1 ] J/K  thermal_time_constant=[ 0 10 ] s  thermal_mass_initial_temperatures=[ 25 25 ] C
  N-Channel MOSFET2 : elec_lib/Semiconductor Devices/N-Channel MOSFET  parameterization=2  prmDatasheet=1  prmEquCoeff=1  Beta=5 A/V^2  Rds=0.025 Ohm  Id=1 A  Vgs=5 V  Vth=0.2 V  lam=0 1/V  Tmeas=25 C  RS=1e-4 Ohm  RD=0.01 Ohm  C_param=1  C_GS=270 pF  C_GD=80 pF  C_iss=350 pF  C_rss=80 pF  dVth_dT=-6 mV/K  Rds_T2=0.037 Ohm  Tmeas2=125 C  BEXDatasheet=-1.5  BEXEquCoeff=-1.5  TdeviceDatasheet=25 C  TdeviceEquCoeff=25 C  LocalVarLogging=[]  Rth=[ 0 10 ] K/W  thermal_mass_parameterization=1  thermal_mass=[ 0 1 ] J/K  thermal_time_constant=[ 0 10 ] s  thermal_mass_initial_temperatures=[ 25 25 ] C
  N-Channel MOSFET3 : elec_lib/Semiconductor Devices/N-Channel MOSFET  parameterization=2  prmDatasheet=1  prmEquCoeff=1  Beta=5 A/V^2  Rds=0.025 Ohm  Id=6 A  Vgs=10 V  Vth=0.2 V  lam=0 1/V  Tmeas=25 C  RS=1e-4 Ohm  RD=0.01 Ohm  C_param=1  C_GS=270 pF  C_GD=80 pF  C_iss=350 pF  C_rss=80 pF  dVth_dT=-6 mV/K  Rds_T2=0.037 Ohm  Tmeas2=125 C  BEXDatasheet=-1.5  BEXEquCoeff=-1.5  TdeviceDatasheet=25 C  TdeviceEquCoeff=25 C  LocalVarLogging=[]  Rth=[ 0 10 ] K/W  thermal_mass_parameterization=1  thermal_mass=[ 0 1 ] J/K  thermal_time_constant=[ 0 10 ] s  thermal_mass_initial_temperatures=[ 25 25 ] C
  Rinduit  6.5 Ohms : fl_lib/Electrical/Electrical Elements/Resistor  Tag=Factory Generic  R=1000 Ohm  i_Log=off  v_Log=off  LocalVarNames=|current|voltage|power  LocalVarDescs=|Resistor current (A)|Voltage across resistor (V)|Power (W)  LocalVarLogging=[0 0 0]
  Rinduit  6.5 Ohms1 : fl_lib/Electrical/Electrical Elements/Resistor  Tag=Factory Generic  R=1000 Ohm  i_Log=off  v_Log=off  LocalVarNames=|current|voltage|power  LocalVarDescs=|Resistor current (A)|Voltage across resistor (V)|Power (W)  LocalVarLogging=[0 0 0]
  Scope  grandeurs électriques : Scope  NumInputPorts=2
  Sonde_I : fl_lib/Electrical/Electrical Sensors/Current Sensor  i1_Log=off  v1_Log=off  LocalVarNames=|i1|v1  LocalVarDescs=|i1|v1  LocalVarLogging=[0 0]
  Sonde_U : fl_lib/Electrical/Electrical Sensors/Voltage Sensor  i1_Log=off  v1_Log=off  LocalVarNames=|i1|v1  LocalVarDescs=|i1|v1  LocalVarLogging=[0 0]
  Switch : fl_lib/Electrical/Electrical Elements/Switch  R_closed=1e-3 Ohm  G_open=1e-4 1/Ohm  Threshold=0.5  i_Log=off  v_Log=off  LocalVarNames=|i|v  LocalVarDescs=|i|v  LocalVarLogging=[0 0]
  Switch1 : fl_lib/Electrical/Electrical Elements/Switch  R_closed=0.001 Ohm  G_open=1e-8 1/Ohm  Threshold=0.5  i_Log=off  v_Log=off  LocalVarNames=|i|v  LocalVarDescs=|i|v  LocalVarLogging=[0 0]
  Verrou : PMIOPort  Port=1  Side=Right
  Déverrou : PMIOPort  Port=2  Side=Left
  M+ : PMIOPort  Port=3  Side=Left
  M- : PMIOPort  Port=4  Side=Left
  +V : PMIOPort  Port=5  Side=Right
  -V : PMIOPort  Port=6  Side=Right
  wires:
  " Conv v"/1 -> Scope  grandeurs électriques/2  "Umoteur"
  " Conv i"/1 -> Scope  grandeurs électriques/1  "Imoteur"
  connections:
  N-Channel MOSFET1/LConn1 -- Switch/LConn1 -- N-Channel MOSFET2/LConn1 -- Rinduit  6.5 Ohms1/LConn1
  Sonde_U/LConn1 -- Sonde_I/LConn1 -- N-Channel MOSFET/RConn1 -- N-Channel MOSFET2/RConn2 -- Diode/LConn1 -- Diode2/RConn1
  Switch1/RConn2 -- Switch/RConn2 -- Diode/RConn1 -- Diode1/RConn1 -- N-Channel MOSFET3/RConn1 -- N-Channel MOSFET2/RConn1 -- +V/RConn1
  M-/RConn1 -- N-Channel MOSFET1/RConn1 -- N-Channel MOSFET3/RConn2 -- Diode3/RConn1 -- Diode1/LConn1 -- Sonde_U/RConn2
  Diode3/LConn1 -- N-Channel MOSFET1/RConn2 -- Rinduit  6.5 Ohms1/RConn1 -- Diode2/LConn1 -- N-Channel MOSFET/RConn2 -- Rinduit  6.5 Ohms/RConn1 -- -V/RConn1
  Sonde_I/RConn1 -- " Conv i"/LConn1
  Sonde_U/RConn1 -- " Conv v"/LConn1
  M+/RConn1 -- Sonde_I/RConn2
  Verrou/RConn1 -- Switch/RConn1
  Déverrou/RConn1 -- Switch1/RConn1
  Switch1/LConn1 -- N-Channel MOSFET/LConn1 -- Rinduit  6.5 Ohms/LConn1 -- N-Channel MOSFET3/LConn1

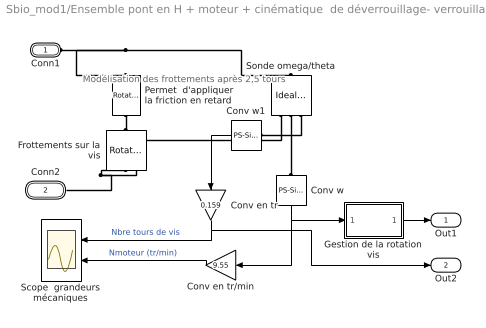
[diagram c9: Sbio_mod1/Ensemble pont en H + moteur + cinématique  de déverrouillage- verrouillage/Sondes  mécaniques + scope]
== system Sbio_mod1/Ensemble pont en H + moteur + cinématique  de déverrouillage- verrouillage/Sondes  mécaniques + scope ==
  note: Modélisation des frottements après 2,5 tours
  Conv en tr : Gain  Gain=0.159
  Conv en tr/min : Gain  Gain=9.55
  Conv w : nesl_utility/PS-Simulink Converter  PhysicalDomain=network_engine_domain  LeftPortType=input  RightPortType=output  SubClassName=ps_output  Unit=1  AffineConversion=off
  Conv w1 : nesl_utility/PS-Simulink Converter  PhysicalDomain=network_engine_domain  LeftPortType=input  RightPortType=output  SubClassName=ps_output  Unit=1  AffineConversion=off
  Frottements sur la vis : fl_lib/Mechanical/Rotational Elements/Rotational Friction  brkwy_trq=2.7e-4 N*m  Col_trq=2.7e-4 N*m  visc_coef=1e-10 N*m/(rad/s)  trans_coef=10 s/rad  vel_thr=10 rad/s  t_Log=off  w_Log=off  LocalVarNames=|t|w  LocalVarDescs=|t|w  LocalVarLogging=[0 0]
  Gestion de la rotation vis : Subsystem
  Permet  d'appliquer la friction en retard : fl_lib/Mechanical/Rotational Elements/Rotational Hard Stop  upper_bnd=2.5 rev  lower_bnd=0 rev  stiff_up=0.2 N*m/rad  stiff_low=0.2 N*m/rad  D_up=0.0026 N*m/(rad/s)  D_low=0.0026 N*m/(rad/s)  initial_angle=0 rad  t_Log=off  w_Log=off  phi_Log=off  LocalVarNames=|t|w|phi  LocalVarDescs=|t|w|phi  LocalVarLogging=[0 0 0]
  Scope  grandeurs mécaniques : Scope  NumInputPorts=2
  Sonde omega/theta : fl_lib/Mechanical/Mechanical Sensors/Ideal Rotational Motion Sensor  offset=0 deg  w_Log=off  t_Log=off  phi_Log=off  LocalVarNames=|w|t|phi  LocalVarDescs=|w|t|phi  LocalVarLogging=[0 0 0]
  Conn1 : PMIOPort  Port=1  Side=Left
  Conn2 : PMIOPort  Port=2  Side=Left
  Out1 : Outport
  Out2 : Outport  Port=2
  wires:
  Conv w1/1 -> Conv en tr/1
  Conv w/1 -> Conv en tr/min/1, Gestion de la rotation vis/1(In1)
  Gestion de la rotation vis/1(Out1) -> Out1/1
  Conv en tr/min/1 -> Scope  grandeurs mécaniques/2  "Nmoteur (tr/min)"
  Conv en tr/1 -> Out2/1, Scope  grandeurs mécaniques/1  "Nbre tours de vis"
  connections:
  Sonde omega/theta/RConn2 -- Conv w/LConn1
  Sonde omega/theta/RConn3 -- Conv w1/LConn1
  Conn1/RConn1 -- Sonde omega/theta/LConn1 -- Permet  d'appliquer la friction en retard/LConn1
  Sonde omega/theta/RConn1 -- Frottements sur la vis/RConn1 -- Conn2/RConn1
  Permet  d'appliquer la friction en retard/RConn1 -- Frottements sur la vis/LConn1

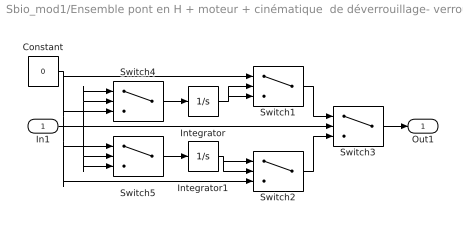
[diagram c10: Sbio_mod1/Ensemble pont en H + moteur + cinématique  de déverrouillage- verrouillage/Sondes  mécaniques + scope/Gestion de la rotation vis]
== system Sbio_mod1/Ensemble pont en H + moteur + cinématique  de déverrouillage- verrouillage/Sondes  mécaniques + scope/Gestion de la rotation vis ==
  In1 : Inport
  Constant : Constant  Value=0
  Integrator : Integrator
  Integrator1 : Integrator
  Switch1 : Switch  Threshold=16.5
  Switch2 : Switch  Threshold=-16.5
  Switch3 : Switch
  Switch4 : Switch
  Switch5 : Switch
  Out1 : Outport
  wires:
  Constant/1 -> Switch1/1, Switch4/3, Switch2/3, Switch5/1
  Switch1/1 -> Switch3/1
  Switch2/1 -> Switch3/3
  Switch4/1 -> Integrator/1
  Integrator/1 -> Switch1/3, Switch1/2
  Switch5/1 -> Integrator1/1
  Integrator1/1 -> Switch2/1, Switch2/2
  In1/1 -> Switch3/2, Switch4/2, Switch4/1, Switch5/2, Switch5/3
  Switch3/1 -> Out1/1
